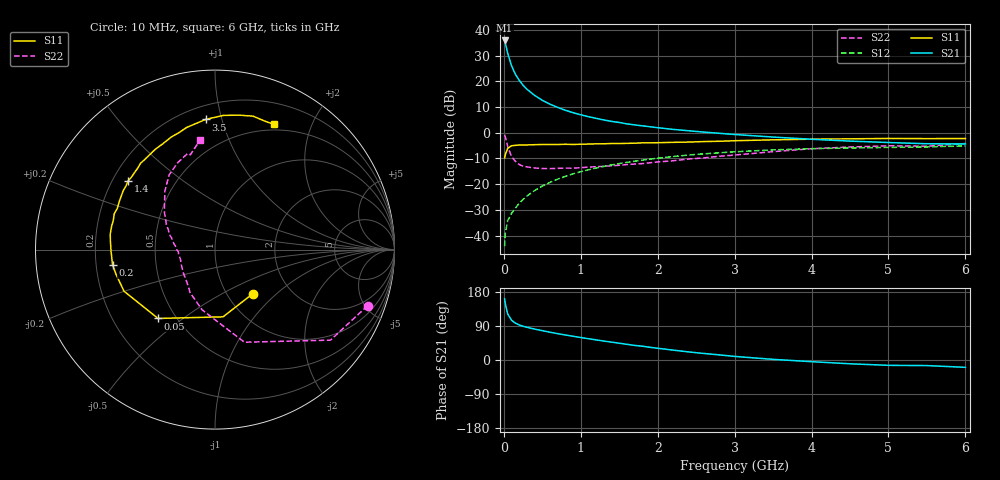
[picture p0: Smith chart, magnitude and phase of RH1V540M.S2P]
! SIEMENS Small Signal Semiconductors
! BFR106
! Si NPN RF Bipolar Junction Transistor in SOT23
! VCE = 1.5 V  IC = 40 mA
! Common Emitter S-Parameters:  August  1996
# GHz  S  MA  R  50
!  f  S11  S21  S12  S22
! GHz  MAG  ANG  MAG  ANG  MAG  ANG  MAG  ANG
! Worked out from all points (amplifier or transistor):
!   36 points, 10 MHz to 6 GHz, reference 50 ohm
!   highest |S21| = 35.9 dB at 10 MHz (marker M1)
!   |S21| within 3 dB of that: start of sweep to 34.67 MHz
!   unconditionally stable (mu >= 1): 241.5 MHz to 2.918 GHz; 4.551 GHz to end of sweep
!   at 250 MHz: K = 1.01, MAG = 21.7 dB, |S12| = -26.0 dB
!   at 1.4 GHz: K = 1.07, MAG = 6.9 dB, |S12| = -12.5 dB
!   at 6 GHz: K = 1.01, MAG = -0.3 dB, |S12| = -5.1 dB
!   S11 on the Smith chart (normalised r, x): 10 MHz: 1.31, -0.72; 50 MHz: 0.40, -0.41; 200 MHz: 0.27, -0.07; 1.4 GHz: 0.26, +0.32; 3.5 GHz: 0.29, +0.89; 6 GHz: 0.43, +1.49
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0.01  0.3236 -49.6  62.44 161.6  0.0062 79.8  0.9057 -20.2
0.02  0.3773 -83.2  55.1 147.3  0.0113 68.1  0.8176 -38.1
0.05  0.4978 -129.6  35.12 121.5  0.0195 55.8  0.5413 -72.4
0.1  0.5574 -155.4  20.08 105.0  0.0269 57.4  0.3435 -102.0
0.15  0.5684 -166.0  13.72 97.2  0.0342 60.7  0.2777 -119.8
0.2  0.5771 -171.6  10.48 92.5  0.0422 63.8  0.2403 -130.6
0.25  0.577 -176.0  8.388 88.9  0.0502 65.7  0.2233 -140.2
0.3  0.5791 -179.0  7.026 86.3  0.0586 67.4  0.2162 -146.0
0.4  0.5848 175.2  5.326 81.6  0.0749 68.8  0.2061 -155.5
0.5  0.59 171.6  4.278 77.4  0.0916 68.7  0.2009 -161.9
0.6  0.5905 167.3  3.587 73.3  0.1081 68.3  0.2001 -166.0
0.8  0.5959 160.5  2.733 66.0  0.1415 66.2  0.2048 -173.3
0.9  0.5906 157.2  2.453 62.6  0.1582 65.0  0.2045 -176.4
1.1  0.6012 150.4  2.053 56.1  0.1901 62.1  0.2144 179.6
1.4  0.6168 141.8  1.662 47.2  0.2363 57.2  0.2273 173.1
1.7  0.6257 133.4  1.42 38.5  0.2789 52.2  0.2456 166.6
2.2  0.6502 120.9  1.162 26.1  0.3444 43.5  0.2844 156.6
3  0.6985 103.1  0.924 9.5  0.4256 30.1  0.3678 140.0
3.5  0.7272 94.1  0.823 1.7  0.4635 22.3  0.4283 130.7
4.5  0.7609 79.9  0.687 -10.0  0.5047 8.2  0.527 113.2
5.5  0.7678 68.6  0.61 -14.7  0.5291 -0.2  0.5458 104.6
6  0.7709 64.8  0.605 -19.4  0.5539 -6.9  0.6161 97.7
